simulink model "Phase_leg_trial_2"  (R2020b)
settings: Solver=FixedStepDiscrete  StartTime=0.0  StopTime=Inf  RelTol=1e-3  EnableMultiTasking=on
model workspace (MAT data in the model file):
  Timer = 3333
  fsw = 15000
undefined symbols (not defined in the file): A, Compare, conversion, DCAEVT1, DCAEVT1FILT, Digital, Down, Event, Filtered, GPTRIP1SEL, GPTRIP2SEL, input, Module, of, start, Trip, TZ1, TZ2, Up, version, Zone
libraries: c2802xlib x1

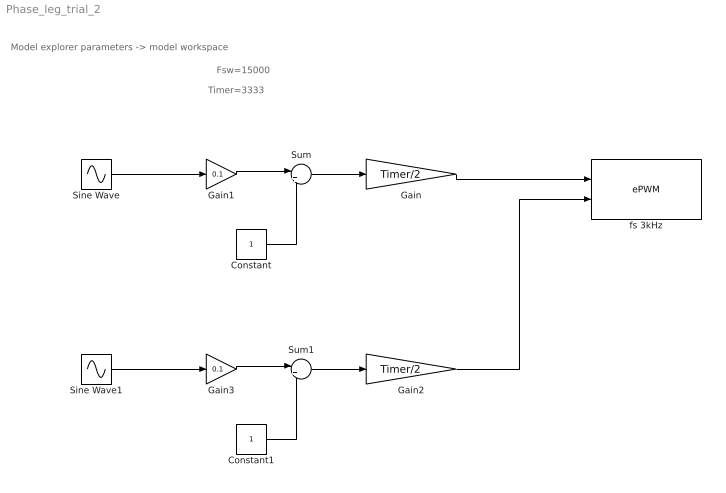
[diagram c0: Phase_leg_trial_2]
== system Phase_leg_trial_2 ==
  note: Model explorer parameters -> model workspace
  note: Timer=3333
  note: Fsw=15000
  Constant : Constant
  Constant1 : Constant
  Gain : Gain  Gain=Timer/2
  Gain1 : Gain  Gain=0.1
  Gain2 : Gain  Gain=Timer/2
  Gain3 : Gain  Gain=0.1
  Sine Wave : Sin  Frequency=100*pi  SampleTime=1/fsw
  Sine Wave1 : Sin  Frequency=100*pi  Phase=pi  SampleTime=1/fsw
  Sum : Sum  Inputs=|++
  Sum1 : Sum  Inputs=|++
  fs 3kHz : c2802xlib/ePWM  PwmType=C2000_Type4  useModule=ePWM1  ePWMxLINKTBPRD=Not Linked  periodUnits=Clock cycles  timerSource=Specify via dialog  timerPeriod_clk=Timer  timerPeriod_sec=1/(2.5e3)  tbshadow=Counter equals to zero  countingMode=Up-Down  phaseActiveEnable=Disable  phaseDirection=Count down after sync  phaseActive=0  synchronizationEnable=off  dcaevt1Sync=off  dcbevt1Sync=off  synchronizationOption=Disable  perSynchronizationOption=Counter equals to period (CTR=PRD)  clockPrescale=1  HSclockPrescale=1  enswap=off  ePWMxAStatus=on  ePWMxAactionLogic1=Do nothing  ePWMxAactionLogic2=Do nothing  ePWMxAactionLogic3=Clear  ePWMxAactionLogic4=Set  ePWMxAactionLogic5=Do nothing  ePWMxAactionLogic6=Do nothing  ePWMxACSFenable=off  ePWMxACSFvalue=Forcing disable  ePWMxASFreload=Zero  ePWMxBStatus=on  ePWMxBactionLogic1=Do nothing  ePWMxBactionLogic2=Do nothing  ePWMxBactionLogic3=Do nothing  ePWMxBactionLogic4=Do nothing  ePWMxBactionLogic5=Clear  ePWMxBactionLogic6=Set  ePWMxBCSFenable=off  ePWMxBCSFvalue=Forcing disable  ePWMxBSFreload=Zero  ePWNxBOutWay=off  ePWMxLINKCMPA=Not Linked  CMPAUnits=Clock cycles  CMPASource=Input port  CMPAValue_per=50  CMPAValue_clk=5e3  enCMPAshadow=Counter equals to zero (CTR=Zero)  ePWMxLINKCMPB=Not Linked  CMPBUnits=Clock cycles  CMPBSource=Input port  CMPBValue_per=50  CMPBValue_clk=5e3  enCMPBshadow=Counter equals to zero (CTR=Zero)  ePWMxLINKCMPC=Not Linked  CMPCUnits=Clock cycles  CMPCSource=Specify via dialog  CMPCValue_per=50  CMPCValue_clk=0  enCMPCshadow=Counter equals to zero (CTR=Zero)  ePWMxLINKCMPD=Not Linked  CMPDUnits=Clock cycles  CMPDSource=Specify via dialog  CMPDValue_per=50  CMPDValue_clk=32000  enCMPDshadow=Counter equals to zero (CTR=Zero)  enableDBePWMxA=on  enableDBePWMxB=on  enhalfcycle=off  DBpolarity=Active high complementary (AHC)  DBedgeDelay=Positive  DBSource_ePWMxA=ePWMxA  DBSource_ePWMxB=ePWMxA  DBPeriodUnits=Clock cycles  DBperiodSource=Specify via dialog  REDperiod=200  FEDperiod=200  REDperiod_sec=0  FEDperiod_sec=0  LoadModeDBRED=Immediate without using shadow  LoadModeDBFED=Immediate without using shadow  adcstartModuleA=on  adcrequestEventA=First event  adcstartEventA=Digital Compare Module A Event 1 start of conversion (DCAEVT1.soc)  adcstartEventA_type2=Counter equals to zero (CTR=Zero)  adcstartModuleB=off  adcrequestEventB=First event  adcstartEventB=Counter equals to zero (CTR=Zero)  adcstartEventB_type2=Counter equals to zero (CTR=Zero)  intEn=off  intPrd=First event  intSel=Counter equals to zero (CTR=Zero)  intSel_type2=Counter equals to zero (CTR=Zero)  hrpe=off  enHRPWM=off  HRPWM_LoadMode=Counter equals to period (CTR=PRD)  HRPWM_CTLMode=Duty or Period control mode  HRPWM_EDGMode=Both edge  hrpeb=off  enHRPWMB=off  HRPWM_LoadModeB=Counter equals to zero (CTR=ZERO)  HRPWM_CTLModeB=Duty or Period control mode  HRPWM_EDGModeB=Both edge  enHRDBRED=off  enHRDBFED=off  enSFO=on  enautoconv=on  chopperEnable=off  chopperFrequency=1  chopperFirstwidth=1  chopperDuty=12.5%  tripZonesource=Specify via dialog  tzselOSHT1=off  tzselOSHT2=off  tzselOSHT3=off  tzselOSHDCAEV1=off  tzselOSHDCBEV1=off  tzselCBC1=off  tzselCBC2=off  tzselCBC3=off  tzselCBCDCAEV2=off  tzselCBCDCBEV2=off  tzselOSHT4=off  tzselOSHT5=off  tzselOSHT6=off  tzselCBC4=off  tzselCBC5=off  tzselCBC6=off  enTzOstIntr=off  enTzCbcIntr=off  enTzDCAEVT1Intr=off  enTzDCAEVT2Intr=off  enTzDCBEVT1Intr=off  enTzDCBEVT2Intr=off  ePWMxAforced=Low  ePWMxBforced=Low  DCAEVT1forced=No action  DCBEVT1forced=No action  DCAEVT2forced=No action  DCBEVT2forced=No action  dcah=Trip Zone 1 input (TZ1)  dcal=Trip Zone 2 input (TZ2)  dcbh=Trip Zone 1 input (TZ1)  dcbl=Trip Zone 2 input (TZ2)  dcah_type2=GPTRIP1SEL/(TZ1)  dcal_type2=GPTRIP2SEL/(TZ2)  dcbh_type2=GPTRIP1SEL/(TZ1)  dcbl_type2=GPTRIP2SEL/(TZ2)  gendcaevt1=Event disabled  gendcaevt2=Event disabled  gendcbevt1=Event disabled  gendcbevt2=Event disabled  dcaevt1src=DCAEVT1 with sync  dcaevt2src=DCAEVT2 with sync  dcbevt1src=DCBEVT1 with sync  dcbevt2src=DCBEVT2 with sync  pulsesel=Counter equals to zero (CTR=Zero)  blankinv=off  blankoffset=0  blankwidth=0  evsrcsel=Filtered version of DCAEVT1 (DCAEVT1FILT)  encape=off
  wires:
  Constant/1 -> Sum/2
  Gain1/1 -> Sum/1
  Sum/1 -> Gain/1
  Sine Wave/1 -> Gain1/1
  Gain/1 -> fs 3kHz/1
  Sum1/1 -> Gain2/1
  Constant1/1 -> Sum1/2
  Sine Wave1/1 -> Gain3/1
  Gain3/1 -> Sum1/1
  Gain2/1 -> fs 3kHz/2
